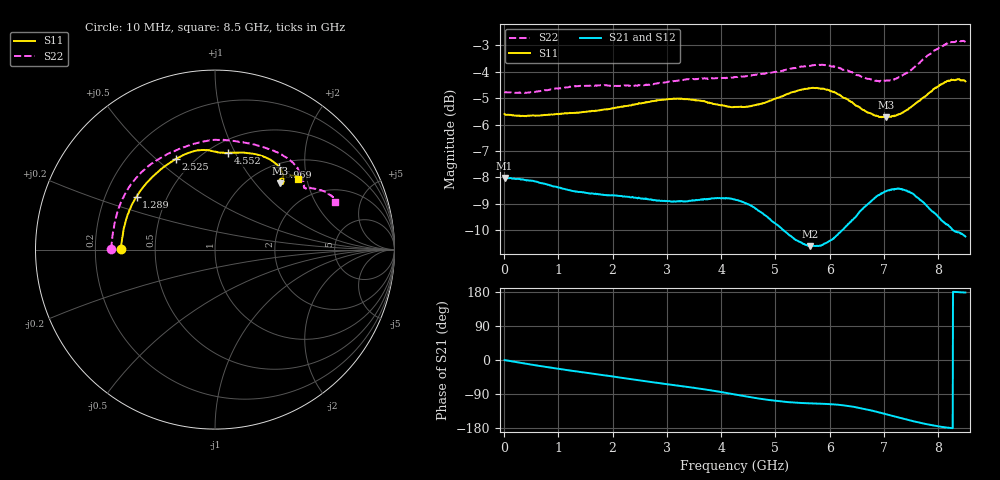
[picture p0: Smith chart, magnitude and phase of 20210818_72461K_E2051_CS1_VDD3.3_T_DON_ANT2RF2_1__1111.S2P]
!Agilent Technologies,E5071C,MY46417908,A.11.23
!Date: Wed Aug 18 14:28:09 2021
!Data & Calibration Information:
!Freq	S11:SOLT2(ON)	S21:SOLT2(ON)	S12:SOLT2(ON)	S22:SOLT2(ON)
!PortZ  Port1:50+j0  Port2:50+j0
!Above PortZ is port z conversion or system Z0 setting when saving the data.
!When reading, reference impedance value at option line is always used.
# Hz S dB R 50
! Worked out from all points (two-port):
!   1601 points, 10 MHz to 8.5 GHz, reference 50 ohm
!   highest |S21| = -8.02 dB at 10 MHz (marker M1); lowest = -10.6 dB at 5.64 GHz (marker M2)
!   |S21| within 3 dB of the highest: start of sweep to end of sweep
!   lowest |S11| = -5.7 dB at 7.035 GHz (marker M3), VSWR 3.14, Z = 67.6 + j68.1 ohm
!   |S11| at or under -10 dB: nowhere
!   |S22| runs from -4.8 to -2.8 dB; largest |S21 - S12| = 0.0014
!   S11 on the Smith chart (normalised r, x): 10 MHz: 0.31, +0.00; 1.289 GHz: 0.34, +0.27; 2.525 GHz: 0.40, +0.58; 4.552 GHz: 0.61, +0.94; 5.969 GHz: 1.05, +1.47; 8.5 GHz: 1.42, +1.76
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1e7  -5.60 179.6  -8.02 -0.4  -8.02 -0.3  -4.75 179.6
7.263438e8  -5.64 161.8  -8.23 -17.4  -8.23 -17.4  -4.71 159.9
1.288806e9  -5.56 145.9  -8.53 -29.3  -8.53 -29.3  -4.55 143.3
1.426769e9  -5.53 141.8  -8.56 -32.0  -8.56 -31.9  -4.53 139.3
1.851269e9  -5.43 129.5  -8.67 -40.4  -8.67 -40.4  -4.51 126.9
2.525162e9  -5.19 113.1  -8.81 -54.3  -8.81 -54.3  -4.51 109.0
2.843538e9  -5.07 106.8  -8.88 -60.7  -8.88 -60.8  -4.43 101.7
3.411306e9  -5.04 97.5  -8.89 -71.7  -8.88 -71.8  -4.27 90.4
4.255e9  -5.33 86.4  -8.84 -91.0  -8.84 -91.0  -4.20 76.8
4.55215e9  -5.30 82.4  -9.08 -98.4  -9.08 -98.3  -4.14 72.4
5.072162e9  -4.96 72.8  -9.87 -108.8  -9.87 -108.8  -3.98 63.6
5.639931e9  -4.62 59.5  -10.61 -114.3  -10.62 -114.2  -3.77 52.9
5.671769e9  -4.61 58.8  -10.60 -114.5  -10.62 -114.4  -3.76 52.2
5.968919e9  -4.69 52.3  -10.45 -116.1  -10.47 -116.2  -3.76 46.7
6.308519e9  -5.02 46.8  -9.84 -120.7  -9.85 -120.9  -3.93 40.6
6.610975e9  -5.44 44.4  -9.19 -128.3  -9.19 -128.3  -4.20 36.8
7.035475e9  -5.72 45.4  -8.53 -142.9  -8.54 -142.9  -4.34 34.5
7.088538e9  -5.70 45.8  -8.49 -145.0  -8.50 -145.0  -4.33 34.4
7.337931e9  -5.54 47.1  -8.45 -154.3  -8.45 -154.3  -4.13 33.5
7.560794e9  -5.23 47.0  -8.67 -162.2  -8.67 -162.3  -3.82 31.9
8.043662e9  -4.48 43.9  -9.59 -176.0  -9.56 -176.0  -3.05 26.4
8.5e9  -4.36 40.5  -10.25 178.0  -10.22 177.9  -2.87 21.8
